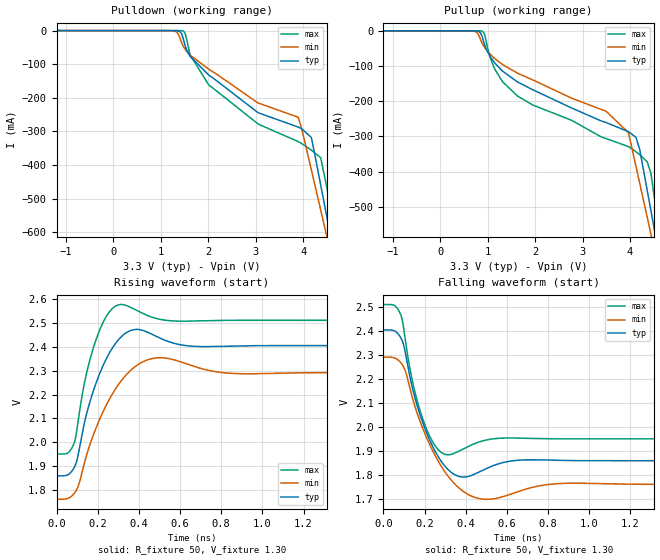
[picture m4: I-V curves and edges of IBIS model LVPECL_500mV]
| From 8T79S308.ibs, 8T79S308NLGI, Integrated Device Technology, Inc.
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[Model]   LVPECL_500mV
Model_type   Output_ECL
Polarity   Non-Inverting
|   typ   min   max
C_comp   2pF   1.5pF   2.5pF
Vmeas= 2.132V
Rref = 50
Cref = 0
Vref = 1.3V
|   typ   min   max
[Voltage range]   3.3V   3.135V   3.465V
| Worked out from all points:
|   rising waveform, R_fixture 50, V_fixture 1.30: 20-80 % time 104ps typ, 138ps min, 79.4ps max; typ from 1.86 V to 2.4 V
|   falling waveform, R_fixture 50, V_fixture 1.30: 20-80 % time 104ps typ, 138ps min, 79.4ps max; typ from 2.4 V to 1.86 V
[Pulldown]
|Voltage   I (typ)   I (min)   I (max)
-1.6V     225.4uA    213.6uA    245.6uA
1.254V    -13.53uA   -453.5uA   -39.94nA
1.467V    -21.75mA   -44.94mA   -1.254mA
1.614V    -76.59mA   -72.83mA   -71.71mA
2.008V    -131.9mA   -114.7mA   -161.4mA
3.058V    -244.8mA   -215.7mA   -278.5mA
3.894V    -287mA     -257.9mA   -330.3mA
4.173V    -317.9mA   -414.4mA   -355.8mA
4.37V     -459.5mA   -533.8mA   -378.3mA
4.517V    -568mA     -624mA     -479.5mA
4.78V     -762.1mA   -785.3mA   -726.3mA
5.944V    -1.337A    -984.5mA   -1.863A
[Pullup]
|Voltage   I (typ)   I (min)   I (max)
-3.3V     763.6uA    674.5uA    902.1uA
679.8mV   -14.22uA   -345.8uA   -69.67nA
877.8mV   -15.09mA   -34.08mA   -1.04mA
1.155V    -92.55mA   -79.71mA   -110.5mA
1.63V     -145.4mA   -120.5mA   -185.5mA
3.491V    -260.3mA   -228mA     -305.9mA
3.967V    -286.5mA   -289.1mA   -328.7mA
4.125V    -302.3mA   -384.8mA   -343.3mA
4.204V    -337.3mA   -432.9mA   -351.9mA
4.442V    -511.6mA   -578.2mA   -405.8mA
5.075V    -982.9mA   -985.2mA   -1.006A
5.947V    -1.332A    -985.2mA   -1.866A
[Ramp]
|   typ   min   max
dV/dt_r   0.367/0.129n   0.355/0.17n   0.375/0.098n
dV/dt_f   0.367/0.129n   0.355/0.17n   0.375/0.098n
R_load =   50.0000
[Rising Waveform]
R_fixture = 50
V_fixture = 1.30   | VCC_typ - 2V
V_fixture_max = 1.465   | VCC_max - 2V
V_fixture_min = 1.135   | VCC_min - 2V
C_fixture = 0.0p
| Time   typ   min   max
0s        1.86V      1.762V     1.951V
84.08ps   1.892V     1.785V     1.993V
136.1ps   2.084V     1.916V     2.251V
182.2ps   2.224V     2.039V     2.404V
240.2ps   2.347V     2.153V     2.524V
298.3ps   2.427V     2.239V     2.575V
384.4ps   2.472V     2.319V     2.554V
496.5ps   2.438V     2.354V     2.516V
858.9ps   2.403V     2.288V     2.51V
2ns       2.405V     2.291V     2.51V
[Falling Waveform]
R_fixture = 50
V_fixture = 1.30   | VCC_typ - 2V
V_fixture_max = 1.465   | VCC_max - 2V
V_fixture_min = 1.135   | VCC_min - 2V
C_fixture = 0.0p
| Time   typ   min   max
0s        2.405V     2.291V     2.51V
84.08ps   2.372V     2.269V     2.468V
136.1ps   2.18V      2.137V     2.211V
182.2ps   2.041V     2.014V     2.057V
240.2ps   1.918V     1.9V       1.937V
298.3ps   1.838V     1.814V     1.887V
384.4ps   1.792V     1.734V     1.907V
496.5ps   1.826V     1.699V     1.946V
858.9ps   1.861V     1.765V     1.951V
2ns       1.86V      1.762V     1.951V
